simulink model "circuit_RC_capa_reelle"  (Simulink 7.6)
settings: Solver=ode15s  StartTime=0.0  StopTime=0.8  RelTol=1e-3
InitFcn:
  | clc
StopFcn:
  | close all
  | load UI_circuit_RC.mat
  | plot(ui(1,:),ui(3,:))
  | hold on
  | plot(ui(1,:),ui(4,:),'r')
  | 
  | title('Tension aux bornes de C idéale et C réelle')
  | xlabel('temps')
  | grid
  | axis([0 0.5 -1 13])
libraries: fl_lib x9, nesl_utility x5, MaLibrairieElectrical_lib x1

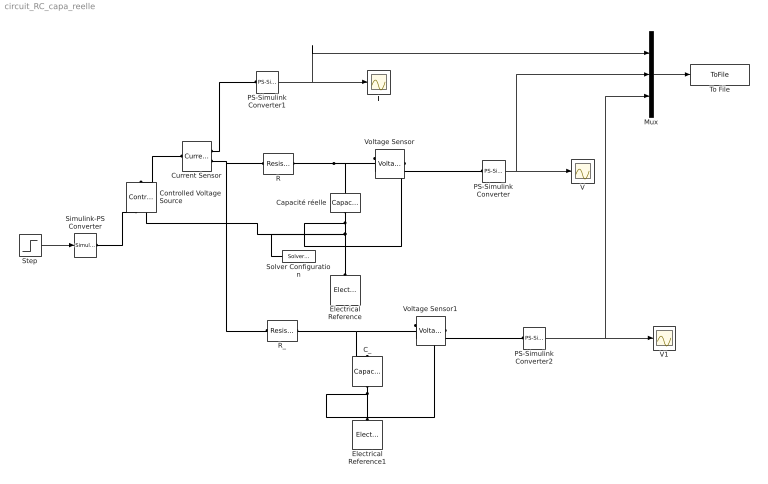
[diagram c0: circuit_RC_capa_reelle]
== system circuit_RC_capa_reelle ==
  C_ : fl_lib/Electrical/Electrical Elements/Capacitor  DialogController=NetworkEngine.DynNeDlgSource  SystemSampleTime=-1  c=1e-3 F  v0=0 V  r=1e-6 Ohm  g=0 1/Ohm  i_Log=off  v_Log=off  vc_Log=off  LocalVarNames=|i|v|vc  LocalVarDescs=|i|v|Internal variable for voltage across capacitor term  LocalVarLogging=[0 0 0]
  Capacité réelle : MaLibrairieElectrical_lib/Capacité réelle  DialogController=NetworkEngine.DynNeDlgSource  SystemSampleTime=-1  C=1e-3 F  v0=0 V  Rs=10 Ohm  Rp=1e+6 Ohm  Ls=1 mH  vc_Log=off  v_Log=off  i_Log=off  LocalVarNames=|vc|v|i  LocalVarDescs=|variable interne qui est la tension aux bornes de la capacité|v|i  LocalVarLogging=[0 0 0]
  Controlled Voltage Source : fl_lib/Electrical/Electrical Sources/Controlled Voltage Source  DialogController=NetworkEngine.DynNeDlgSource  SystemSampleTime=-1  i_Log=off  v_Log=off  LocalVarNames=|i|v  LocalVarDescs=|i|v  LocalVarLogging=[0 0]
  Current Sensor : fl_lib/Electrical/Electrical Sensors/Current Sensor  DialogController=NetworkEngine.DynNeDlgSource  SystemSampleTime=-1  i1_Log=off  v1_Log=off  LocalVarNames=|i1|v1  LocalVarDescs=|i1|v1  LocalVarLogging=[0 0]
  Electrical Reference : fl_lib/Electrical/Electrical Elements/Electrical Reference  DialogController=NetworkEngine.DynNeDlgSource  SystemSampleTime=-1  i_Log=off  LocalVarNames=|i  LocalVarDescs=|i  LocalVarLogging=0
  Electrical Reference1 : fl_lib/Electrical/Electrical Elements/Electrical Reference  DialogController=NetworkEngine.DynNeDlgSource  SystemSampleTime=-1  i_Log=off  LocalVarNames=|i  LocalVarDescs=|i  LocalVarLogging=0
  I : Scope
  Mux : Mux  Inputs=3
  PS-Simulink Converter : nesl_utility/PS-Simulink Converter  DialogController=NetworkEngine.DynNeUtilDlgSource  SystemSampleTime=-1  PhysicalDomain=network_engine_domain  LeftPortType=input  RightPortType=output  SubClassName=ps_output  Unit=1  AffineConversion=off
  PS-Simulink Converter1 : nesl_utility/PS-Simulink Converter  DialogController=NetworkEngine.DynNeUtilDlgSource  SystemSampleTime=-1  PhysicalDomain=network_engine_domain  LeftPortType=input  RightPortType=output  SubClassName=ps_output  Unit=1  AffineConversion=off
  PS-Simulink Converter2 : nesl_utility/PS-Simulink Converter  DialogController=NetworkEngine.DynNeUtilDlgSource  SystemSampleTime=-1  PhysicalDomain=network_engine_domain  LeftPortType=input  RightPortType=output  SubClassName=ps_output  Unit=1  AffineConversion=off
  R : fl_lib/Electrical/Electrical Elements/Resistor  DialogController=NetworkEngine.DynNeDlgSource  SystemSampleTime=-1  R=0.1 kOhm  i_Log=off  v_Log=off  LocalVarNames=|i|v  LocalVarDescs=|i|v  LocalVarLogging=[0 0]
  R_ : fl_lib/Electrical/Electrical Elements/Resistor  DialogController=NetworkEngine.DynNeDlgSource  SystemSampleTime=-1  R=0.1 kOhm  i_Log=off  v_Log=off  LocalVarNames=|i|v  LocalVarDescs=|i|v  LocalVarLogging=[0 0]
  Simulink-PS Converter : nesl_utility/Simulink-PS Converter  DialogController=NetworkEngine.DynNeUtilDlgSource  SystemSampleTime=-1  PhysicalDomain=network_engine_domain  LeftPortType=input  RightPortType=output  SubClassName=ps_input  Unit=1  AffineConversion=off  InputFilterTimeConstant=.001  UdotUserProvided=0
  Solver Configuration : nesl_utility/Solver Configuration  DialogController=NetworkEngine.DynNeUtilDlgSource  SystemSampleTime=-1  PhysicalDomain=network_engine_domain  LeftPortType=input  RightPortType=generic  SubClassName=solver  Accelerate=off  Profile=off  ResidualTolerance=1e-9  MaxNonlinIter=3  MaxModeIter=2  DoFixedCost=off  UseLocalSampling=off  DoDC=off  LinearAlgebra=Sparse  LocalSolverSampleTime=.001  LocalSolverChoice=NE_BACKWARD_EULER_ADVANCER  UseLocalSolver=off
  Step : Step  Time=0  After=12  SampleTime=0
  To File : ToFile  Filename=UI_circuit_RC  MatrixName=ui
  V : Scope
  V1 : Scope
  Voltage Sensor : fl_lib/Electrical/Electrical Sensors/Voltage Sensor  DialogController=NetworkEngine.DynNeDlgSource  SystemSampleTime=-1  i1_Log=off  v1_Log=off  LocalVarNames=|i1|v1  LocalVarDescs=|i1|v1  LocalVarLogging=[0 0]
  Voltage Sensor1 : fl_lib/Electrical/Electrical Sensors/Voltage Sensor  DialogController=NetworkEngine.DynNeDlgSource  SystemSampleTime=-1  i1_Log=off  v1_Log=off  LocalVarNames=|i1|v1  LocalVarDescs=|i1|v1  LocalVarLogging=[0 0]
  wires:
  Step/1 -> Simulink-PS Converter/1
  PS-Simulink Converter/1 -> V/1, Mux/2
  PS-Simulink Converter1/1 -> I/1, Mux/1
  Mux/1 -> To File/1
  PS-Simulink Converter2/1 -> Mux/3, V1/1
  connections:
  Capacité réelle/RConn1 -- Controlled Voltage Source/RConn2 -- Solver Configuration/RConn1 -- Electrical Reference/LConn1 -- Voltage Sensor/RConn2
  R/RConn1 -- Voltage Sensor/LConn1 -- Capacité réelle/LConn1
  Simulink-PS Converter/RConn1 -- Controlled Voltage Source/RConn1
  Voltage Sensor/RConn1 -- PS-Simulink Converter/LConn1
  Current Sensor/LConn1 -- Controlled Voltage Source/LConn1
  Current Sensor/RConn1 -- PS-Simulink Converter1/LConn1
  Current Sensor/RConn2 -- R/LConn1 -- R_/LConn1
  R_/RConn1 -- C_/LConn1 -- Voltage Sensor1/LConn1
  C_/RConn1 -- Electrical Reference1/LConn1 -- Voltage Sensor1/RConn2
  Voltage Sensor1/RConn1 -- PS-Simulink Converter2/LConn1
